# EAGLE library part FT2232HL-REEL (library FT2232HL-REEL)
FTDI Chip FT2232HL-REEL, USB Controller, 4-channel, 480MBps, USB 2.0, 64-Pin LQFP Source: Datasheet
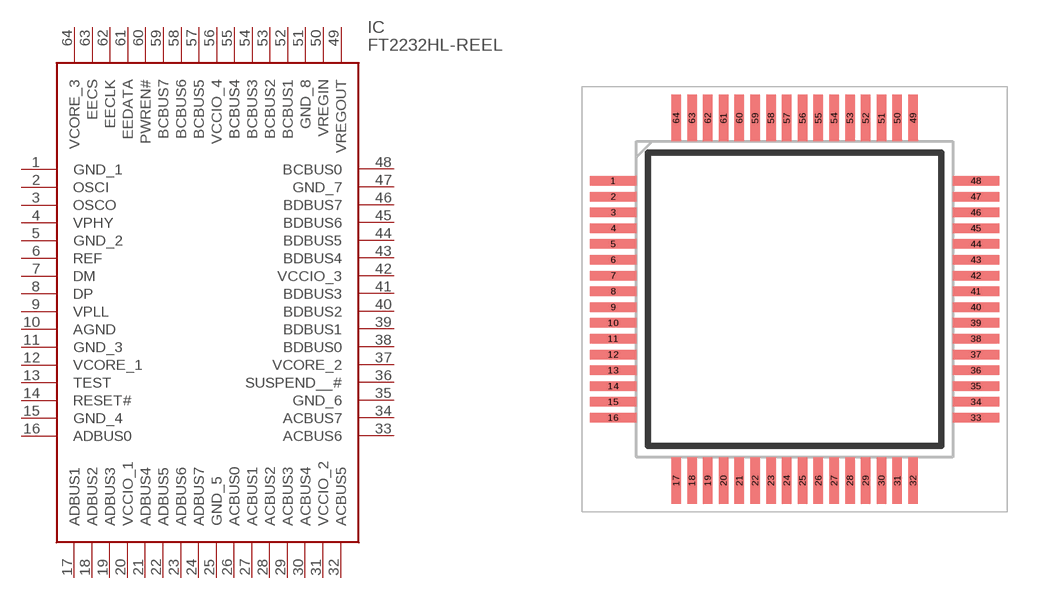
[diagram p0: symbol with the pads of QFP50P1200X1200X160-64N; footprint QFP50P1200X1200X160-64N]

Designator prefix IC

## FT2232HL-REEL (Description: FTDI Chip FT2232HL-REEL, USB Controller, 4-channel, 480MBps, USB 2.0, 64-Pin LQFP; Height: 1.6mm; Manufacturer_Name: FTDI Chip; Manufacturer_Part_Number: FT2232HL-REEL; Mouser_Part_Number: 895-FT2232HL; Mouser_Price-Stock: https://www.mouser.co.uk/ProductDetail/FTDI/FT2232HL-REEL?qs=D1%2FPMqvA100v7FHcEx164g%3D%3D)  [QFP50P1200X1200X160-64N]
1  GND_1
2  OSCI
3  OSCO
4  VPHY
5  GND_2
6  REF
7  DM
8  DP
9  VPLL
10  AGND
11  GND_3
12  VCORE_1
13  TEST
14  RESET#
15  GND_4
16  ADBUS0
17  ADBUS1
18  ADBUS2
19  ADBUS3
20  VCCIO_1
21  ADBUS4
22  ADBUS5
23  ADBUS6
24  ADBUS7
25  GND_5
26  ACBUS0
27  ACBUS1
28  ACBUS2
29  ACBUS3
30  ACBUS4
31  VCCIO_2
32  ACBUS5
33  ACBUS6
34  ACBUS7
35  GND_6
36  SUSPEND__#
37  VCORE_2
38  BDBUS0
39  BDBUS1
40  BDBUS2
41  BDBUS3
42  VCCIO_3
43  BDBUS4
44  BDBUS5
45  BDBUS6
46  BDBUS7
47  GND_7
48  BCBUS0
49  VREGOUT
50  VREGIN
51  GND_8
52  BCBUS1
53  BCBUS2
54  BCBUS3
55  BCBUS4
56  VCCIO_4
57  BCBUS5
58  BCBUS6
59  BCBUS7
60  PWREN#
61  EEDATA
62  EECLK
63  EECS
64  VCORE_3

## Footprint QFP50P1200X1200X160-64N (pad centres in mm)
LQFP-64
smd 1.475 x 0.3: 1 -5.738,3.75; 2 -5.738,3.25; 3 -5.738,2.75; 4 -5.738,2.25; 5 -5.738,1.75; 6 -5.738,1.25; 7 -5.738,0.75; 8 -5.738,0.25; 9 -5.738,-0.25; 10 -5.738,-0.75; 11 -5.738,-1.25; 12 -5.738,-1.75; 13 -5.738,-2.25; 14 -5.738,-2.75; 15 -5.738,-3.25; 16 -5.738,-3.75; 33 5.738,-3.75; 34 5.738,-3.25; 35 5.738,-2.75; 36 5.738,-2.25; 37 5.738,-1.75; 38 5.738,-1.25; 39 5.738,-0.75; 40 5.738,-0.25; 41 5.738,0.25; 42 5.738,0.75; 43 5.738,1.25; 44 5.738,1.75; 45 5.738,2.25; 46 5.738,2.75; 47 5.738,3.25; 48 5.738,3.75
smd 0.3 x 1.475: 17 -3.75,-5.738; 18 -3.25,-5.738; 19 -2.75,-5.738; 20 -2.25,-5.738; 21 -1.75,-5.738; 22 -1.25,-5.738; 23 -0.75,-5.738; 24 -0.25,-5.738; 25 0.25,-5.738; 26 0.75,-5.738; 27 1.25,-5.738; 28 1.75,-5.738; 29 2.25,-5.738; 30 2.75,-5.738; 31 3.25,-5.738; 32 3.75,-5.738; 49 3.75,5.738; 50 3.25,5.738; 51 2.75,5.738; 52 2.25,5.738; 53 1.75,5.738; 54 1.25,5.738; 55 0.75,5.738; 56 0.25,5.738; 57 -0.25,5.738; 58 -0.75,5.738; 59 -1.25,5.738; 60 -1.75,5.738; 61 -2.25,5.738; 62 -2.75,5.738; 63 -3.25,5.738; 64 -3.75,5.738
